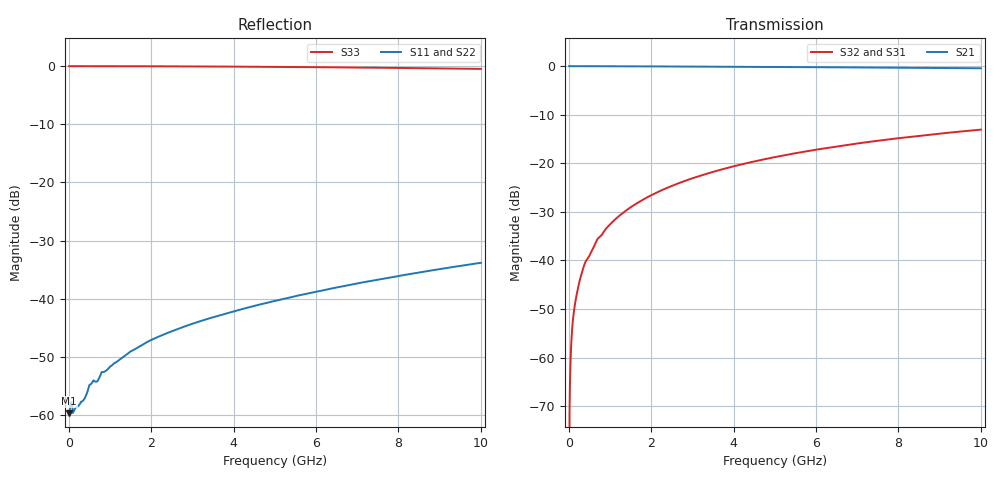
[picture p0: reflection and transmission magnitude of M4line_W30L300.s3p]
! Created Fri Sep 09 14:26:39 2011
# hz S ma R 50
! 3 Port Network Data from SP1.SP block
! freq  magS11  angS11  magS12  angS12  magS13  angS13
!  magS21  angS21
!  magS22  angS22  magS23  angS23
!  magS31  angS31  magS32  angS32
!  magS33  angS33
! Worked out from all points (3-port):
!   1000 points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, 10 MHz to 10 GHz, reference 50 ohm
!   strongest paths, dB at 10 MHz, 2.51 GHz, 5.01 GHz, 7.51 GHz, 10 GHz:
!     S21: 0.0, -0.1, -0.2, -0.3, -0.4
!     S32: -, -24.6, -18.7, -15.4, -13.1
!     S31: -, -24.6, -18.7, -15.4, -13.1
!   lowest |S11| = -59.7 dB at 10 MHz (marker M1), VSWR 1.00, Z = 50.1 + j0.014 ohm
!   |S11| at or under -10 dB: start of sweep to end of sweep
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1e7  0.001035 7.7  0.999 -0.0  0 0.0
     0.999 -0.0  0.001035 7.7  0 0.0
     0 0.0  0 0.0  1 0.0
8e7  0.001255 4.1  0.9987 -0.1  0.001867 89.8
     0.9987 -0.1  0.001255 4.1  0.001867 89.8
     0.001867 89.8  0.001867 89.8  1 -0.2
1.2e8  0.001078 7.5  0.9989 -0.2  0.00284 89.8
       0.9989 -0.2  0.001078 7.5  0.00284 89.8
       0.00284 89.8  0.00284 89.8  1 -0.3
1.7e8  0.00116 9.5  0.9988 -0.2  0.00394 89.7
       0.9988 -0.2  0.00116 9.5  0.00394 89.7
       0.00394 89.7  0.00394 89.7  1 -0.5
3.7e8  0.00136 21.4  0.9987 -0.5  0.008777 89.2
       0.9987 -0.5  0.00136 21.4  0.008777 89.2
       0.008777 89.2  0.008777 89.2  0.9999 -1.0
7.2e8  0.002017 26.8  0.9979 -1.0  0.01697 88.5
       0.9979 -1.0  0.002017 26.8  0.01697 88.5
       0.01697 88.5  0.01697 88.5  0.9997 -1.9
1.36e9  0.003229 16.2  0.9958 -1.9  0.03187 87.1
        0.9958 -1.9  0.003229 16.2  0.03187 87.1
        0.03187 87.1  0.03187 87.1  0.9988 -3.7
2.24e9  0.004819 -5.4  0.9924 -3.0  0.05241 85.5
        0.9924 -3.0  0.004819 -5.4  0.05241 85.5
        0.05241 85.5  0.05241 85.5  0.9972 -6.0
5.01e9  0.00959 -56.1  0.9801 -6.2  0.1159 79.9
        0.9801 -6.2  0.00959 -56.1  0.1159 79.9
        0.1159 79.9  0.1159 79.9  0.9861 -13.4
1e10  0.02036 -107.5  0.9504 -11.5  0.2221 70.3
      0.9504 -11.5  0.02036 -107.5  0.2221 70.3
      0.2221 70.3  0.2221 70.3  0.9476 -26.2
